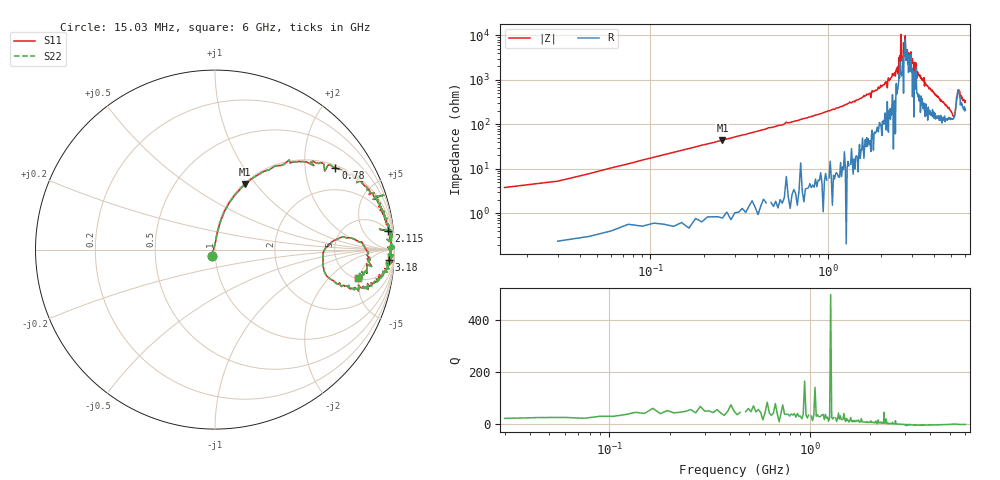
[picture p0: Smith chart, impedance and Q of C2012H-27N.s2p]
!	Network	Analyzer	HP8753E.07.74:	Oct	30	2002	Serial	No.	JP38451487
!	Hewlett-Packard
!	28	Aug	2009	9:58:33
!	Frequency	S11	S21	S12	S22
#	HZ	S	RI	R	50
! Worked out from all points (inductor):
!   400 points, 15.03 MHz to 6 GHz, reference 50 ohm
!   read as one part in series: L = 27.5 nH near 45.03 MHz
!   highest Q = 50 at 255 MHz (marker M1), where L = 27.7 nH
!   self-resonance near 2.775 GHz
!   S11 on the Smith chart (normalised r, x): 15.03 MHz: 0.96, -0.07; 780 MHz: 1.08, +2.88; 2.115 GHz: 5, +17; 3.18 GHz: 14, -27; 6 GHz: 5.15, -4.83
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1.502992e7  -0.0171 -0.0342  1.02 0.0342  1.02 0.0342  -0.0171 -0.0342
9.002955e7  0.0289 0.152  0.971 -0.152  0.971 -0.152  0.0289 0.152
2.550287e8  0.169 0.366  0.831 -0.366  0.831 -0.366  0.169 0.366
7.800261e8  0.671 0.457  0.329 -0.457  0.329 -0.457  0.671 0.457
1.020025e9  0.794 0.389  0.206 -0.389  0.206 -0.389  0.794 0.389
2.01002e9  0.964 0.135  0.0363 -0.135  0.0363 -0.135  0.964 0.135
2.115019e9  0.966 0.105  0.0341 -0.105  0.0341 -0.105  0.966 0.105
2.505017e9  0.958 0.0569  0.0419 -0.0569  0.0419 -0.0569  0.958 0.0569
2.535017e9  0.986 0.0275  0.014 -0.0275  0.014 -0.0275  0.986 0.0275
2.580017e9  0.98 0.0315  0.0197 -0.0315  0.0197 -0.0315  0.98 0.0315
2.595017e9  0.999 0.00952  0.00137 -0.00952  0.00137 -0.00952  0.999 0.00952
2.610017e9  0.981 0.0298  0.0193 -0.0298  0.0193 -0.0298  0.981 0.0298
2.685017e9  0.999 0.0147  0.00131 -0.0147  0.00131 -0.0147  0.999 0.0147
2.730016e9  0.979 0.00787  0.0209 -0.00787  0.0209 -0.00787  0.979 0.00787
2.745016e9  0.992 0.00595  0.00836 -0.00595  0.00836 -0.00595  0.992 0.00595
2.775016e9  0.97 0.0126  0.0301 -0.0126  0.0301 -0.0126  0.97 0.0126
3.015015e9  0.994 -0.0328  0.00574 0.0328  0.00574 0.0328  0.994 -0.0328
3.180014e9  0.968 -0.0558  0.0315 0.0558  0.0315 0.0558  0.968 -0.0558
4.00501e9  0.915 -0.17  0.0851 0.17  0.0851 0.17  0.915 -0.17
5.010005e9  0.676 -0.184  0.324 0.184  0.324 0.184  0.676 -0.184
5.445003e9  0.855 -0.0196  0.145 0.0196  0.145 0.0196  0.855 -0.0196
6e9  0.799 -0.158  0.201 0.158  0.201 0.158  0.799 -0.158
